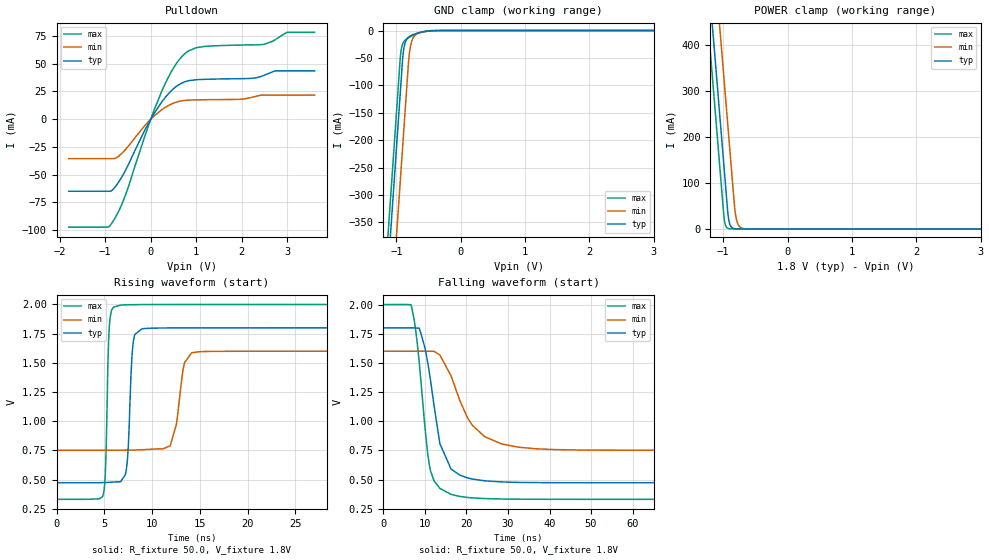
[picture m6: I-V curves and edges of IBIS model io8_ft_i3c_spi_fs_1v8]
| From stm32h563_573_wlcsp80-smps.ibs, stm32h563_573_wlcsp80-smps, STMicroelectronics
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[Model]   io8_ft_i3c_spi_fs_1v8
Model_type I/O_open_drain
Polarity   Non-Inverting
Enable   Active-Low
| CAP_THRESHOLD on pad IOFT is "UDTCAPC" :
| Rising=20.0% of vddiom   Falling=80.0% of vddiom
| C_comp min and max val. don't necessarily correlate with the min and max pvt
| but are the smallest and greatest pad capacitance found.
| var   typ   min   max
C_comp   3.75301pF  3.69047pF  3.87697pF
|C_comp_pulldown   3.75301pF  3.69047pF  3.87697pF
Vinl = 800.0mV
Vinh = 1.0V
Vmeas = 900.0mV   | Reference voltage for timing measurements
Cref  = 50.0pF   | Timing specification test load capacitance value
Rref  = 1.0MOhm   | Timing specification test load resistance value
Vref  = 990.0mV   | Timing specification test load voltage
[Model Spec]
| TIME_THRESHOLD on pin ZII2CV11 is "CMOS" :
| Rising=40.0% of vdd   Falling=60.0% of vdd
Vinl 703.80000mV 631.80000mV 784.80000mV
Vinh 1.06220V 937.20000mV 1.16620V
| variable   typ   min   max
[Temperature Range] 25.0 125.0 -40.0
| variable   typ   min   max
[Voltage Range] 1.8V 1.6V 2.0V
| variable   typ   min   max
[POWER Clamp Reference] 1.8V 1.6V 2.0V
| variable   typ   min   max
[GND Clamp Reference] 0V 0V 0V
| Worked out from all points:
|   slope of the pulldown table from 0 to 0.27 V, typ, clamps not added: 15.8 ohm
|   GND clamp passes 1 mA (typ) near -0.52 V on its own axis
|   POWER clamp passes 1 mA (typ) near -0.84 V on its own axis
|   rising waveform, R_fixture 50.0, V_fixture 1.8V: 20-80 % time 403ps typ, 865ps min, 285ps max; typ from 0.474 V to 1.8 V
|   falling waveform, R_fixture 50.0, V_fixture 1.8V: 20-80 % time 3.95ns typ, 7.1ns min, 2.73ns max; typ from 1.8 V to 0.474 V
[POWER Clamp]
-1.8V     1.518A     1.709A     1.407A
-1.23V    548.8mA    740.2mA    437.5mA
-1.16V    429.8mA    621.2mA    318.5mA
-1.05V    242.8mA    434.2mA    131.5mA
-980mV    123.8mA    315.2mA    17.95mA
-930mV    38.81mA    230.2mA    1.49mA
-910mV    17.82mA    196.2mA    550.8uA
-890mV    8.18mA     162.2mA    203.5uA
-810mV    363.5uA    33.6mA     3.797uA
-770mV    76.62uA    10.47mA    518.8nA
-710mV    7.416uA    1.822mA    26.34nA
3.6V      0A         0A         0A
[GND Clamp]
-1.8V     -1.579A    -1.74A     -1.515A
-1.24V    -627.3mA   -788.3mA   -562.7mA
-1.05V    -304.3mA   -465.3mA   -239.7mA
-940mV    -117.3mA   -278.3mA   -52.69mA
-930mV    -100.3mA   -261.3mA   -40.52mA
-900mV    -50.11mA   -210.3mA   -24.23mA
-880mV    -30.95mA   -176.3mA   -20.02mA
-810mV    -12.18mA   -57.97mA   -13.23mA
-780mV    -9.807mA   -29.1mA    -11.19mA
-690mV    -5.41mA    -7.142mA   -6.184mA
-420mV    -170.4uA   -446.1uA   -81.94uA
3.6V      5.755nA    953.4nA    228.2pA
| variable   typ   min   max
[Pullup Reference] 1.8V 1.6V 2.0V
| variable   typ   min   max
[Pulldown Reference] 0V 0V 0V
[Pulldown]
-1.8V     -65.02mA   -35.56mA   -97.42mA
-940mV    -65.02mA   -35.56mA   -97.42mA
-850mV    -64.17mA   -35.56mA   -93.49mA
-570mV    -47.32mA   -28.01mA   -70.04mA
-120mV    -9.088mA   -5.279mA   -14.07mA
250mV     16.04mA    8.832mA    26.05mA
520mV     28.19mA    14.82mA    47.53mA
780mV     34.17mA    17.07mA    60.14mA
1.18V     35.97mA    17.56mA    65.65mA
2.49V     39.57mA    21.77mA    67.55mA
2.99V     43.62mA    21.77mA    78.38mA
3.6V      43.62mA    21.77mA    78.38mA
[Ramp]
dV/dt_r 795.76131mV/399.73992ps 508.933mV/787.83421ps 1.00097V/282.8293ps
dV/dt_f 795.78722mV/3.5588ns 508.9803mV/6.69308ns 1.00099V/2.73063ns
R_load = 50.0
| Removed startup time: 0s 0s 0s  .
| Removed end time: 36.4ns.
[Rising Waveform]
R_fixture   = 50.0
V_fixture   = 1.8V
V_fixture_min = 1.6V
V_fixture_max = 2.0V
0s        473.7mV    751.7mV    331.7mV
4.9ns     475mV      751.6mV    375.3mV
5.5ns     477.4mV    751.8mV    1.773V
5.95ns    479.7mV    751.8mV    1.977V
7.25ns    559.8mV    752.2mV    1.997V
8ns       1.656V     753.3mV    1.998V
8.95ns    1.792V     756.2mV    1.999V
11.9ns    1.799V     790mV      2V
14.15ns   1.8V       1.587V     2V
36.4ns    1.8V       1.6V       2V
| Removed startup time: 0s 0s 0s  .
| Removed end time: 199.4ns.
[Falling Waveform]
R_fixture   = 50.0
V_fixture   = 1.8V
V_fixture_min = 1.6V
V_fixture_max = 2.0V
0s        1.8V       1.6V       2V
6.65ns    1.8V       1.6V       1.996V
8.7ns     1.789V     1.6V       1.475V
10.2ns    1.593V     1.6V       880mV
11.25ns   1.374V     1.6V       590.8mV
13.6ns    808.1mV    1.568V     425.1mV
16.3ns    590.9mV    1.389V     374mV
21.45ns   505.2mV    964.7mV    344mV
32.55ns   476.7mV    778.2mV    332.9mV
199.4ns   473.7mV    751.7mV    331.7mV
